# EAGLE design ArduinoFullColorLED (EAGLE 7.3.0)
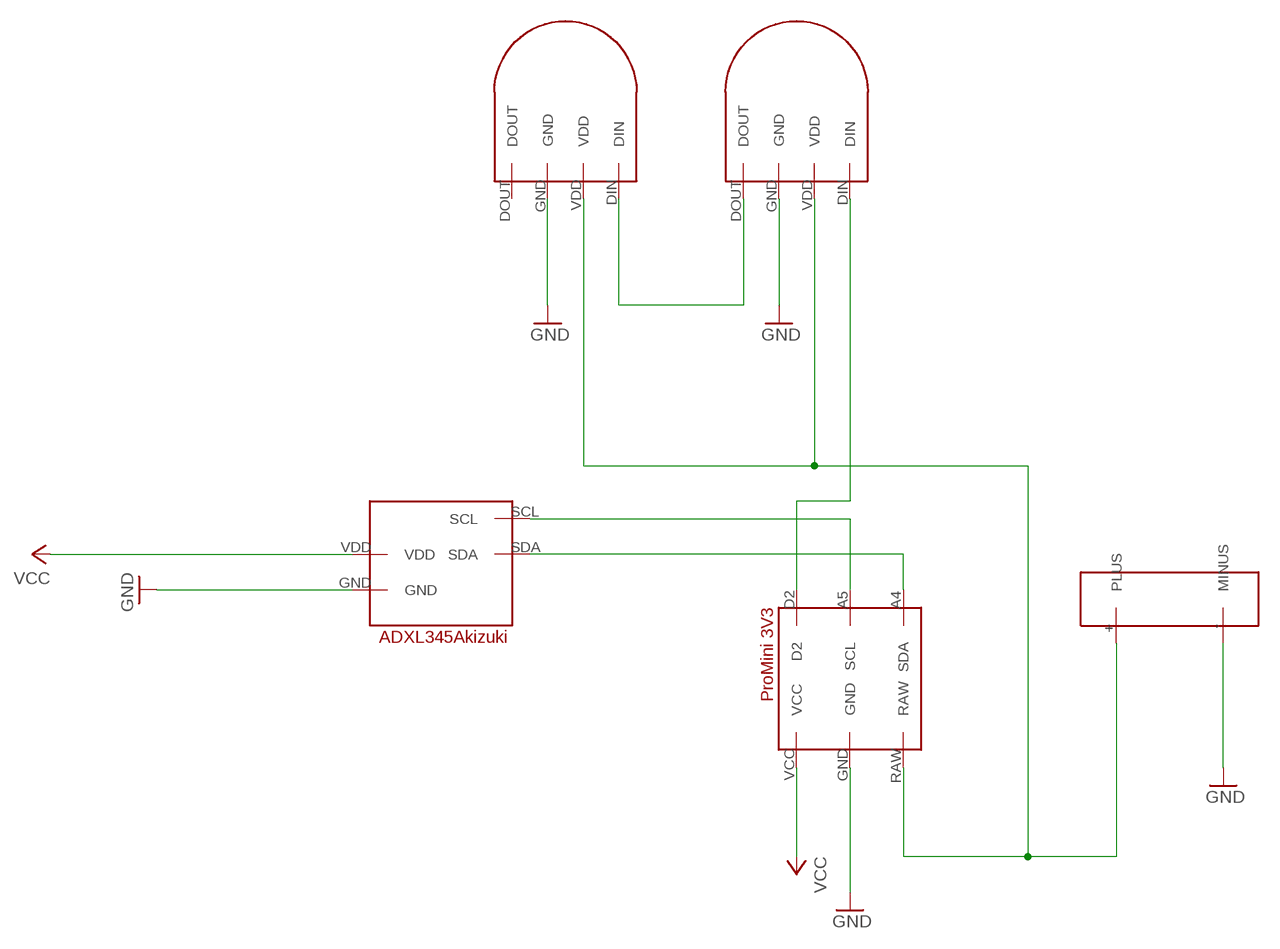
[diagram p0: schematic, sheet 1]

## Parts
U$1  ADXL345AKIZUKI  [ADXL345AKIZUKI]
U$2  CR2032BOX  [CR2032BOX]
U$3  ARDUINOPROMINI_VBTECH  [ARDUINOPROMINI_VBTECH]
U$4  RGBLED_PL9823F5  [RGBLED_PL9823F5]
U$5  RGBLED_PL9823F5  [RGBLED_PL9823F5]

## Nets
GND: U$1.GND U$2.-(MINUS) U$3.GND U$4.GND U$5.GND
N$1: U$3.D2 U$5.DIN
N$2: U$1.SDA U$3.A4(SDA)
N$4: U$4.DIN U$5.DOUT
N$9: U$1.SCL U$3.A5(SCL)
N$10: U$2.+(PLUS) U$3.RAW U$4.VDD U$5.VDD
VCC: U$1.VDD U$3.VCC
Unconnected: U$4.DOUT

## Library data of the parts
U$1 = VBTechLibs:ADXL345AKIZUKI: ADXL345 Accelerometer Module
U$2 = VBTechLibs:CR2032BOX: CR2032BOX
U$3 = VBTechLibs:ARDUINOPROMINI_VBTECH: Arduino Pro Mini 3.3V
U$4 U$5 = VBTechLibs:RGBLED_PL9823F5: RGBLED PL9823

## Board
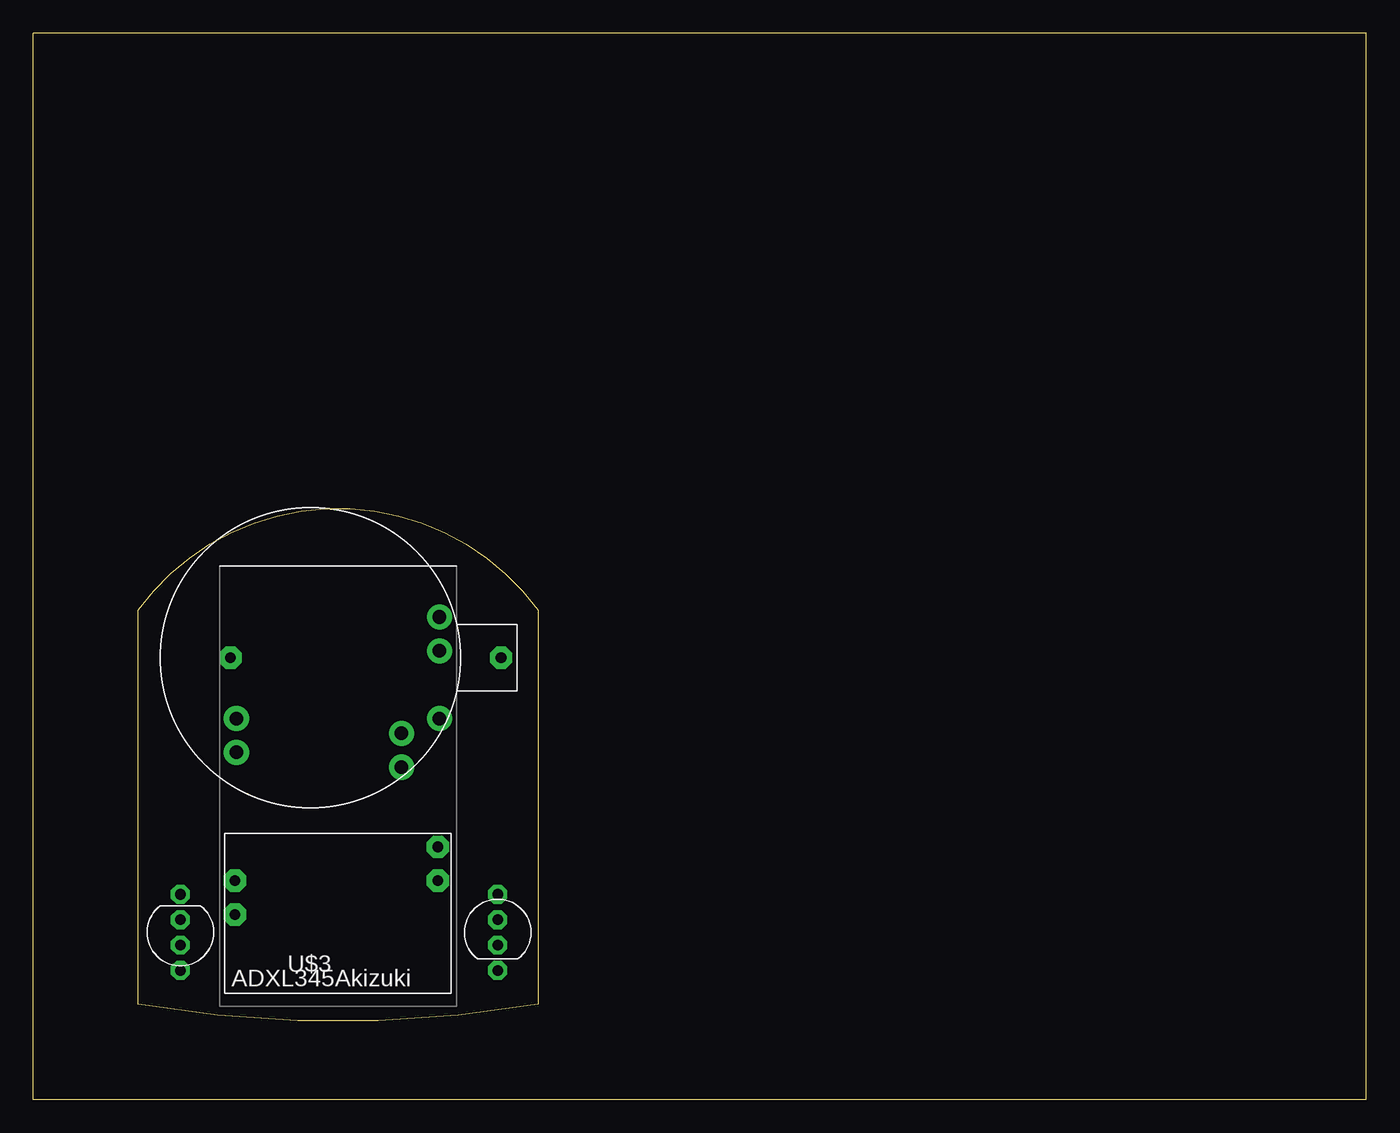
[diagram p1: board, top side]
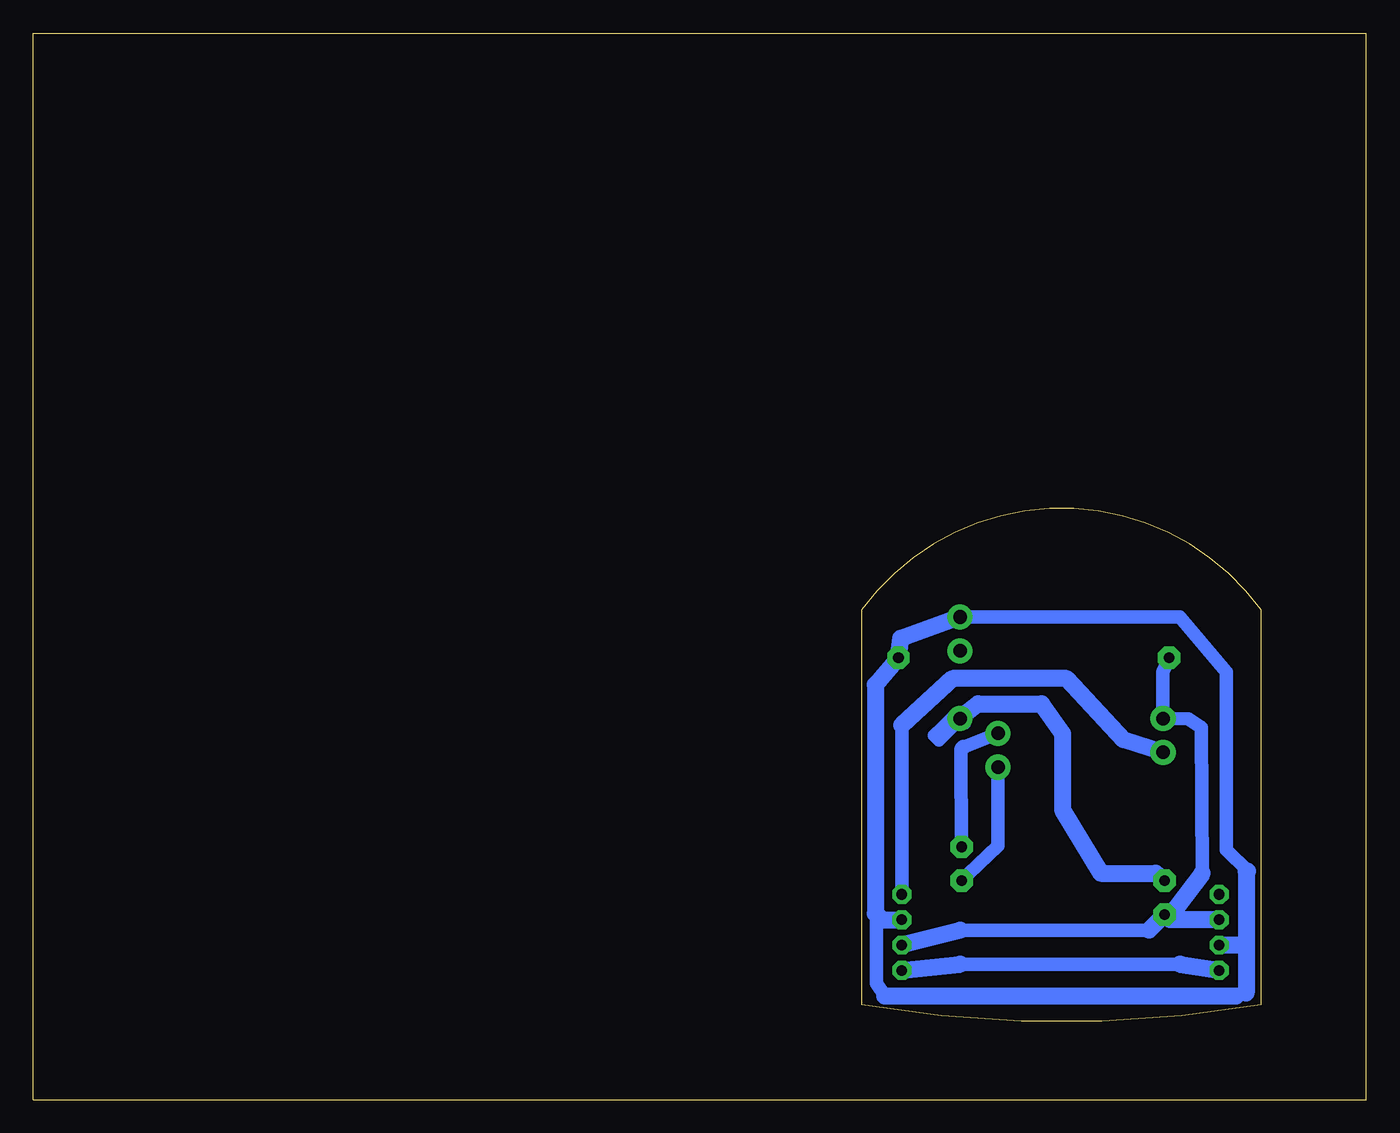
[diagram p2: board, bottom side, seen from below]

Size 100.01 x 80.01 mm. Coordinates in mm from the lower left corner, seen from the top.
Outline: 100,0 100,80 0,80
Outline: 100.01,0 0,0 0,80.01
Outline: 7.86,36.75 arc-108 37.86,36.75 37.86,7.14 arc-20 7.86,7.14 7.86,36.75
Copper layers (1*16): Top 0.035mm / dielectric 1.5mm / Bottom 0.035mm
Design rules "default": minimum track width 10mil, minimum drill 24mil, track to track 8mil, track to pad 8mil, pad to pad 8mil, via to via 8mil, smd to smd 8mil, copper to edge 40mil, drill to drill 8mil, minimum pad ring 10mil, minimum via ring 8mil, stop-mask expansion 4mil, vias tented up to drill 0mil, thermal gap 10mil

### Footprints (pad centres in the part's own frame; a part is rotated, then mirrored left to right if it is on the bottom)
ADXL345AKIZUKI = drill 0.8 pad 1.676 octagon: GND -15.24,-5.08; SCL 0,0; SDA 0,-2.54; VDD -15.24,-2.54
CR2032BOX = drill 0.8 pad 1.676 octagon: + 25.32,0; - 5,0
ARDUINOPROMINI_VBTECH = drill 1.016 pad 1.88: A4 4.763,1.429; A5 4.763,3.969; D2 -7.62,2.54; GND -7.62,5.08; GND2 7.62,10.16; RAW 7.62,12.7; VCC 7.62,5.08
RGBLED_PL9823F5 = drill 0.8 pad 1.422 octagon: DIN 2.857,0; DOUT -2.857,0; GND -0.953,0; VDD 0.953,0

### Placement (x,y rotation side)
U$1  30.36,18.96 0 top
U$2  9.78,33.15 0 top
U$3  22.86,23.51 0 top
U$4  11.04,12.54 270 top
U$5  34.85,12.54 90 top

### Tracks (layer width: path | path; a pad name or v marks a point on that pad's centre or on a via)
GND
  Bottom 1.016: 12.3,16.99 12.38,27.94 13.34,28.57 U$3.GND 15.24,32.07 U$2.- | 14.21,14.45 14.92,13.97 U$1.GND 14.73,13.49 | 16.3,12.7 30.48,12.7
  Bottom 1.27: 12.3,16.99 14.21,14.45 | U$4.GND 14.73,13.49 | U$1.GND 16.3,12.7 | 30.48,12.7 U$5.GND
N$1
  Bottom 1.016: 34.85,28.1 U$5.DIN
  Bottom 1.27: U$3.D2 18.19,27 22.46,31.59 31.04,31.59 34.85,28.1
N$2
  Bottom 1.016: U$1.SDA 29.83,16.92 27.62,19.05 27.62,25.08 arc-21 U$3.A4
N$4
  Bottom 1.016: 30.48,10.16 13.97,10.16
  Bottom 1.27: U$5.DOUT 30.48,10.16 | 13.97,10.16 U$4.DIN
N$9
  Bottom 1.016: U$1.SCL 30.4,26.2 arc90 30.09,26.51 U$3.A5
N$10
  Bottom 1.016: U$5.VDD 35.16,13.49 | 36.75,13.89 36.75,8.73 36.12,7.78 | 8.89,17.14 10.48,18.73 10.48,32.07 13.97,36.2 U$3.RAW
  Bottom 1.27: 36.12,7.78 9.77,7.78 | U$3.RAW 34.92,34.61 U$2.+ 36.83,31.11 36.83,13.97 36.75,13.89 36.35,13.49 U$5.VDD | 8.89,17.14 9,17.14 9,11.59 | 9,11.59 9,8 | U$4.VDD 9,11.59
N$13
  Bottom 1.016: 30.48,28.57 31.43,27.62 | 31.43,27.62 31.75,27.94 | 31.75,27.94 30.8,28.89 30.48,28.57 | 30.16,28.26 30.48,28.57 | 31.43,27.62 32.07,26.99 32.38,27.3 31.75,27.94
VCC
  Bottom 1.27: U$3.VCC 30.16,28.89 29.13,29.69 24.37,29.69 22.78,27.46 22.78,21.75 19.93,16.99 15.82,16.99 U$1.VDD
